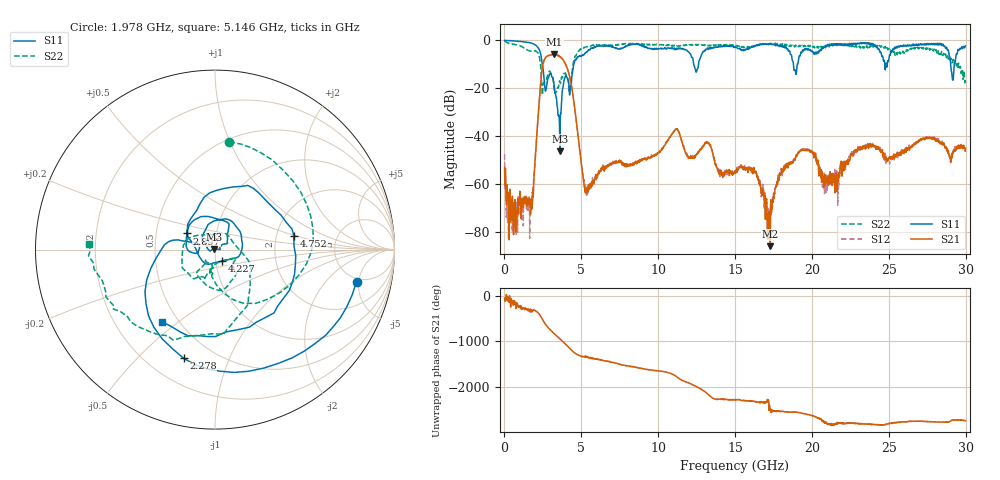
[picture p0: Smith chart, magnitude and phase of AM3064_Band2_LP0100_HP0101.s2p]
# Hz S DB R 50.0
!freq dBS11 angS11 dBS21 angS21 dBS12 angS12 dBS22 angS22
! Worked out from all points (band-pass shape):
!   1600 points, 10 MHz to 29.98 GHz, reference 50 ohm
!   highest |S21| = -5.88 dB at 3.234 GHz (marker M1); lowest = -86.0 dB at 17.29 GHz (marker M2)
!   |S21| within 3 dB of the highest: 2.551 GHz to 3.892 GHz (1.341 GHz wide, 41.6 % of centre)
!   lowest |S11| = -46.3 dB at 3.609 GHz (marker M3), VSWR 1.01, Z = 49.7 + j0.337 ohm
!   |S11| at or under -10 dB: 2.457 GHz to 4.508 GHz (2.051 GHz wide, 58.9 % of centre); 12.31 GHz to 12.62 GHz (307.4 MHz wide, 2.47 % of centre); 18.8 GHz to 19.05 GHz (250.5 MHz wide, 1.32 % of centre)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
!   |S22| runs from -22.8 to -0.2 dB; largest |S21 - S12| = 0.014
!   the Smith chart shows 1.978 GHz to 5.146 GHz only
!   S11 on the Smith chart (normalised r, x): 1.978 GHz: 4.53, -4.66; 2.278 GHz: 0.34, -0.69; 2.897 GHz: 0.72, +0.13; 4.227 GHz: 1.08, -0.14; 4.752 GHz: 2.51, +0.47; 5.146 GHz: 0.41, -0.44
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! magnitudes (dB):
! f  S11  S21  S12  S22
! 10 MHz  0.0  -53.1  -47.6  -0.2
! 647.3 MHz  -0.3  -72.2  -74.6  -1.7
! 1.641 GHz  -1.0  -67.2  -82.7  -4.5
! 1.978 GHz  -1.8  -51.6  -51.6  -4.4
! 2.278 GHz  -4.0  -24.1  -24.2  -7.2
! 2.897 GHz  -14.9  -6.3  -6.3  -13.1
! 3.234 GHz  -19.0  -5.9  -5.9  -20.8
! 3.609 GHz  -46.3  -6.9  -6.7  -17.2
! 4.227 GHz  -22.5  -14.8  -14.7  -20.7
! 4.752 GHz  -7.0  -37.8  -37.9  -5.2
! 5.015 GHz  -6.7  -52.0  -52.4  -3.7
! 5.146 GHz  -6.1  -59.0  -59.0  -3.1
! 10 GHz  -3.5  -46.9  -46.7  -1.8
! 11.2 GHz  -3.6  -37.0  -36.9  -2.3
! 15 GHz  -2.6  -54.6  -55.1  -1.9
! 16.28 GHz  -2.3  -55.2  -54.6  -2.4
! 17.29 GHz  -1.7  -86.0  -73.0  -1.4
! 18.06 GHz  -2.1  -55.0  -56.6  -1.8
! 19.99 GHz  -4.3  -46.8  -47.1  -2.2
! 20.91 GHz  -2.1  -59.5  -63.7  -2.7
! 25 GHz  -8.0  -49.4  -49.6  -3.4
! 29.98 GHz  -2.3  -46.3  -46.0  -15.8
